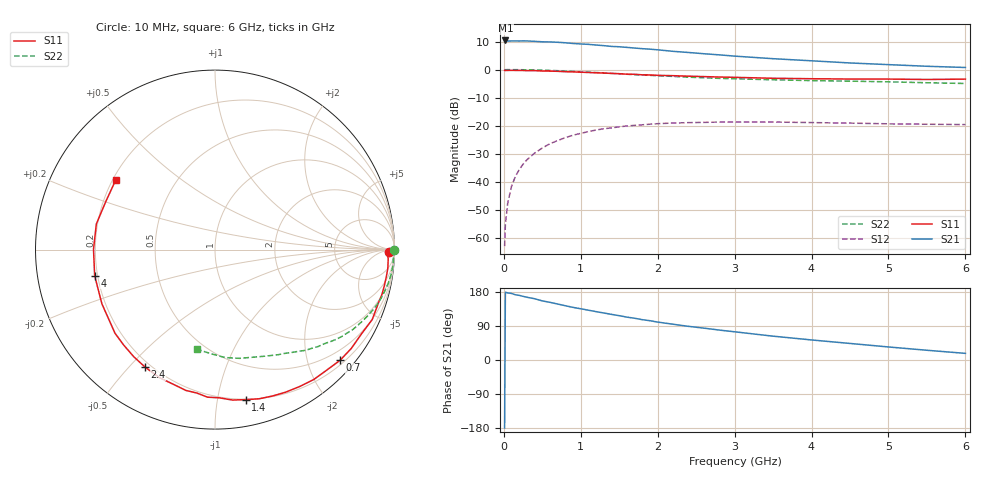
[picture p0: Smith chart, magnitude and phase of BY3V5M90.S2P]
! SIEMENS Small Signal Semiconductors
! BFY420
! Si NPN RF SIEGET Grounded Emitter Transistor in MICRO-X
! VCE = 3.5 V  IC = 0.9 mA
! Common Emitter S-Parameters:  October  1996
# GHz  S  MA  R  50
!  f  S11  S21  S12  S22
! GHz  MAG  ANG  MAG  ANG  MAG  ANG  MAG  ANG
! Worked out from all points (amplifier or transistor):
!   36 points, 10 MHz to 6 GHz, reference 50 ohm
!   highest |S21| = 10.4 dB at 20 MHz (marker M1)
!   |S21| within 3 dB of that: start of sweep to 1.836 GHz
!   unconditionally stable (mu >= 1): 4.546 GHz to end of sweep
!   at 250 MHz: K = 0.04, MSG = 22.0 dB, |S12| = -33.8 dB
!   at 1.4 GHz: K = 0.18, MSG = 14.6 dB, |S12| = -20.8 dB
!   at 6 GHz: K = 1.35, MAG = 6.7 dB, |S12| = -19.7 dB
!   S11 on the Smith chart (normalised r, x): 10 MHz: 52, -22; 700 MHz: 0.28, -2.61; 1.4 GHz: 0.20, -1.20; 2.4 GHz: 0.18, -0.55; 4 GHz: 0.19, -0.10; 6 GHz: 0.21, +0.30
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0.01  0.9678 -0.8  3.307 -179.4  0.0007 81.0  0.9999 -0.2
0.02  0.9606 -1.4  3.311 178.8  0.0017 94.7  0.9932 -0.5
0.05  0.9664 -3.1  3.239 177.1  0.0041 79.3  0.9977 -1.3
0.1  0.9686 -6.3  3.241 175.6  0.0082 87.9  0.9949 -2.8
0.15  0.9662 -9.2  3.244 172.1  0.0123 83.0  0.9955 -4.2
0.2  0.9647 -12.2  3.238 170.6  0.0163 82.3  0.9947 -5.5
0.3  0.9579 -18.0  3.246 165.6  0.0244 79.0  0.99 -8.3
0.4  0.9588 -24.0  3.193 161.7  0.0322 75.5  0.9836 -11.0
0.5  0.9412 -30.1  3.134 156.0  0.0397 71.7  0.974 -13.7
0.7  0.9307 -41.5  3.073 147.7  0.054 65.0  0.9535 -18.8
0.9  0.9093 -52.7  2.923 138.8  0.0672 58.0  0.9263 -23.6
1.1  0.8864 -63.7  2.82 131.4  0.078 52.0  0.8985 -28.3
1.4  0.8531 -78.5  2.591 120.4  0.0908 43.7  0.8557 -34.5
1.8  0.8056 -97.2  2.361 106.4  0.1031 34.0  0.7989 -41.5
2.2  0.7776 -113.5  2.117 94.4  0.1109 25.7  0.7551 -48.0
2.4  0.7617 -120.8  2.019 88.8  0.1127 22.6  0.7311 -50.9
2.8  0.7357 -133.9  1.831 79.0  0.1153 16.6  0.6961 -56.2
3.5  0.6988 -154.4  1.564 62.9  0.1154 8.9  0.6566 -64.7
4  0.686 -167.8  1.434 52.9  0.113 5.0  0.6349 -70.9
4.5  0.6769 179.8  1.312 43.7  0.1104 2.1  0.6211 -77.3
5.5  0.6647 156.1  1.145 25.7  0.1055 0.9  0.5812 -92.0
6  0.6756 144.9  1.089 17.5  0.104 2.0  0.5641 -100.3
